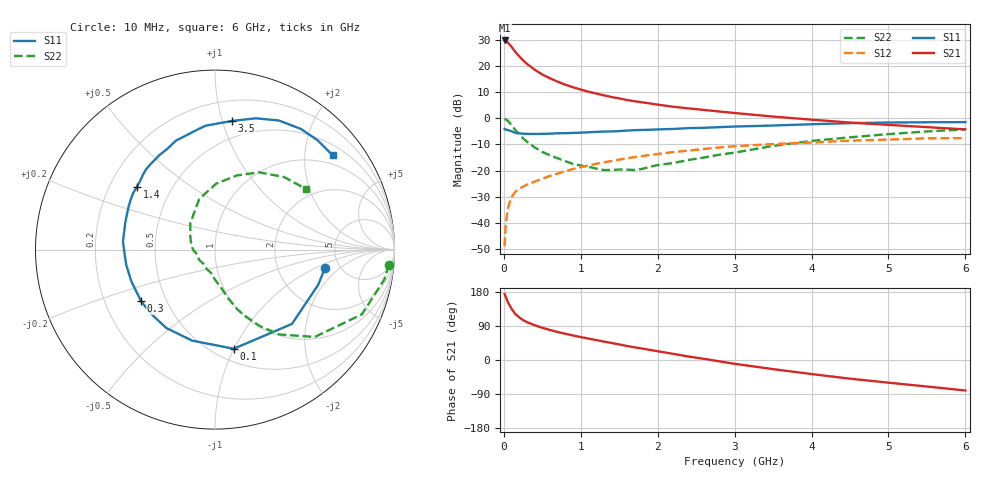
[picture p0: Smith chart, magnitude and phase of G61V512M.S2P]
! SIEMENS Small Signal Semiconductors
! BFG193
! Si NPN RF Bipolar Junction Transistor in SOT223
! VCE = 1.5 V  IC = 12 mA
! Common Emitter S-Parameters:  August  1996
# GHz  S  MA  R  50
!  f  S11  S21  S12  S22
! GHz  MAG  ANG  MAG  ANG  MAG  ANG  MAG  ANG
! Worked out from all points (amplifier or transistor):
!   36 points, 10 MHz to 6 GHz, reference 50 ohm
!   highest |S21| = 29.7 dB at 10 MHz (marker M1)
!   |S21| within 3 dB of that: start of sweep to 114.6 MHz
!   unconditionally stable (mu >= 1): 788.6 MHz to 2.779 GHz
!   at 250 MHz: K = 0.60, MSG = 24.1 dB, |S12| = -26.2 dB
!   at 1.4 GHz: K = 1.07, MAG = 10.6 dB, |S12| = -16.4 dB
!   at 6 GHz: K = 0.94, MSG = 1.7 dB, |S12| = -7.6 dB
!   S11 on the Smith chart (normalised r, x): 10 MHz: 3.84, -1.27; 100 MHz: 0.62, -1.00; 300 MHz: 0.36, -0.28; 1.4 GHz: 0.32, +0.32; 3.5 GHz: 0.36, +1.08; 6 GHz: 0.75, +2.66
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0.01  0.6218 -9.4  30.44 174.2  0.0036 88.4  0.9729 -5.0
0.02  0.6075 -18.8  30.1 169.6  0.0076 84.3  0.9581 -10.0
0.05  0.5961 -44.0  27.91 153.6  0.0185 71.9  0.8943 -23.8
0.1  0.5621 -79.3  23.02 135.4  0.0313 60.2  0.7387 -41.2
0.15  0.5229 -104.1  18.36 121.2  0.0394 53.0  0.5928 -52.9
0.2  0.5143 -121.8  15.16 112.4  0.0447 51.1  0.4929 -59.7
0.25  0.5048 -134.9  12.69 105.3  0.0491 49.3  0.4101 -65.3
0.3  0.5023 -145.0  10.89 99.9  0.0536 49.3  0.357 -69.4
0.4  0.4986 -159.2  8.433 91.9  0.0616 49.6  0.2767 -75.3
0.5  0.5018 -170.2  6.819 84.9  0.0699 50.0  0.2267 -79.5
0.6  0.5052 -178.3  5.761 79.3  0.0791 50.6  0.1953 -84.0
0.7  0.515 174.8  4.972 73.9  0.0878 50.9  0.1715 -89.1
0.8  0.5158 168.5  4.35 69.2  0.0973 50.1  0.1505 -94.2
1.1  0.5375 153.7  3.205 56.5  0.1249 48.0  0.1181 -112.8
1.4  0.5582 141.1  2.529 44.9  0.1521 43.4  0.1022 -137.4
1.7  0.5893 130.7  2.103 33.4  0.1803 38.6  0.1025 -162.8
2.2  0.6219 115.1  1.654 16.3  0.2246 28.3  0.139 164.0
2.8  0.6729 99.1  1.339 -3.5  0.2758 15.3  0.2006 133.4
3.5  0.7235 82.4  1.072 -24.1  0.32 -1.3  0.2953 107.3
4.5  0.8025 63.7  0.825 -49.3  0.372 -20.8  0.4306 73.6
5.5  0.8354 46.8  0.674 -70.0  0.4134 -43.8  0.5582 46.4
6  0.8401 38.7  0.611 -80.4  0.4166 -56.9  0.6104 33.5
